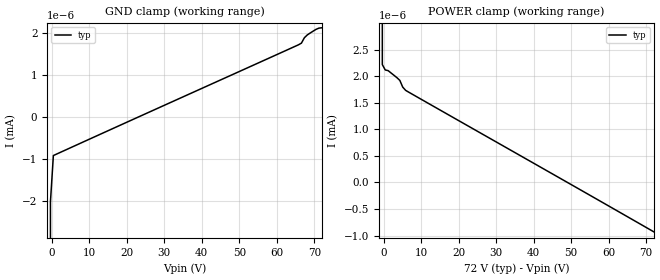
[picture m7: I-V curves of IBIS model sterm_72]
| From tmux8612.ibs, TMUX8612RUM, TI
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| sterm_72
[Model]   sterm_72
Model_type   Terminator
|   typ   min   max
C_comp   1.008417e-11   NA   NA
[Voltage Range]   72   NA   NA
[Temperature Range]   27   NA   NA
[Power Clamp Reference]   72   NA   NA
[GND Clamp Reference]   0   NA   NA
[GND Clamp]
|   Voltage   I(typ)   I(min)   I(max)
-5V       -2.416A    NA         NA
-1.111V   -48.55mA   NA         NA
-333.3mV  -2.008nA   NA         NA
444.4mV   -911.8pA   NA         NA
65.78V    1.717nA    NA         NA
66.56V    1.757nA    NA         NA
67.33V    1.884nA    NA         NA
68.11V    1.951nA    NA         NA
70.44V    2.083nA    NA         NA
72V       2.121nA    NA         NA
[POWER Clamp]
|   Voltage   I(typ)   I(min)   I(max)
-5V       1.055A     NA         NA
-1.111V   25.66mA    NA         NA
-333.3mV  2.217nA    NA         NA
444.4mV   2.116nA    NA         NA
1.222V    2.103nA    NA         NA
4.333V    1.919nA    NA         NA
5.111V    1.792nA    NA         NA
5.889V    1.731nA    NA         NA
72V       -929.9pA   NA         NA
